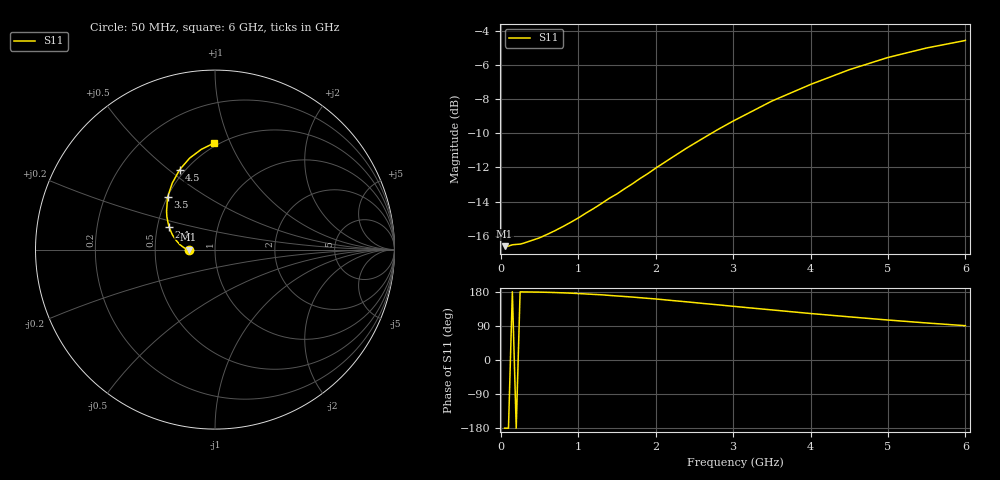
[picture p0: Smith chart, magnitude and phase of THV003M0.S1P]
! SIEMENS Discrete & RF Semiconductors
! BAS70
! Si Schottky Diode in SOT23
! IF = 3 mA
! S-Parameters:  February  1997
# GHz  S  MA  R  50
!  f  S11
! GHz  MAG  ANG
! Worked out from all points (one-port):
!   34 points, 50 MHz to 6 GHz, reference 50 ohm
!   lowest |S11| = -16.6 dB at 50 MHz (marker M1), VSWR 1.35, Z = 37.1 - j0.0195 ohm
!   |S11| at or under -10 dB: start of sweep to 2.718 GHz
!   S11 on the Smith chart (normalised r, x): 50 MHz: 0.74, -0.00; 2.4 GHz: 0.58, +0.16; 3.5 GHz: 0.50, +0.35; 4.5 GHz: 0.47, +0.55; 6 GHz: 0.48, +0.87
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0.05  0.1475 -179.9
0.1  0.1475 -180.0
0.15  0.1489 180.0
0.25  0.1495 179.9
0.3  0.1506 179.6
0.5  0.156 179.1
0.7  0.1638 178.0
0.8  0.1683 177.3
1  0.1784 175.4
1.3  0.1968 172.1
1.4  0.2038 170.5
1.5  0.21 169.0
1.6  0.2175 167.6
1.7  0.2249 166.1
1.8  0.2332 164.4
1.9  0.2411 162.7
2  0.25 161.1
2.2  0.2676 157.2
2.4  0.2863 153.5
2.6  0.3049 149.5
2.8  0.3244 145.7
3  0.3438 141.7
3.5  0.3936 132.2
4  0.4405 122.7
4.5  0.4868 113.9
5  0.5289 105.5
5.5  0.564 97.7
6  0.5934 90.5
